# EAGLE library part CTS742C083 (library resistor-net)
Chip Resistor Array 4 Single Resistor Source: http://www.ctscorp.com/components/Datasheets/CTSChipArrayDs.pdf
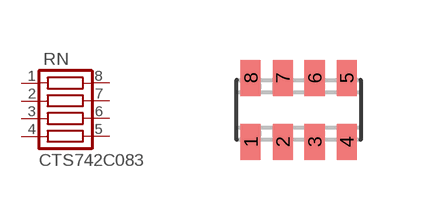
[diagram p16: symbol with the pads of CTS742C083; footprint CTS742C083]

Designator prefix RN

## CTS742C083 (OC_FARNELL: unknown; OC_NEWARK: unknown)  [CTS742C083]
1  1  pas
2  2  pas
3  3  pas
4  4  pas
5  5  pas
6  6  pas
7  7  pas
8  8  pas

## Footprint CTS742C083 (pad centres in mm)
Chip Resistor Array Source: http://www.ctscorp.com/components/Datasheets/CTSChipArrayDs.pdf
smd 0.5 x 0.9: 1 -1.2,-0.8; 2 -0.4,-0.8; 3 0.4,-0.8; 4 1.2,-0.8; 5 1.2,0.8; 6 0.4,0.8; 7 -0.4,0.8; 8 -1.2,0.8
